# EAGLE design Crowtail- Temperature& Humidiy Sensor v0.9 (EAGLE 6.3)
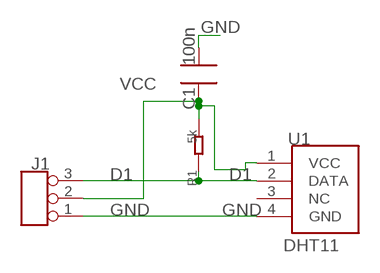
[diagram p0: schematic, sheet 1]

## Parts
C1  100n  C0603  [0603]
J1  TINKER_3P_DIP  [3P_2.0_DIP]
R1  5k  R0603  [0603]
U1  DHT11  [DHT11]

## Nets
D1: J1.3 R1.1 U1.2(DATA)
GND: C1.2 J1.1 U1.4(GND)
VCC: C1.1 J1.2 R1.2 U1.1(VCC)
Unconnected: U1.3(NC)

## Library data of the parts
C1 = CPT_SMD:C0603; C0603: 100N
J1 = Connector:TINKER_3P_DIP
R1 = CPT_SMD:R0603
U1 = Sensors:DHT11

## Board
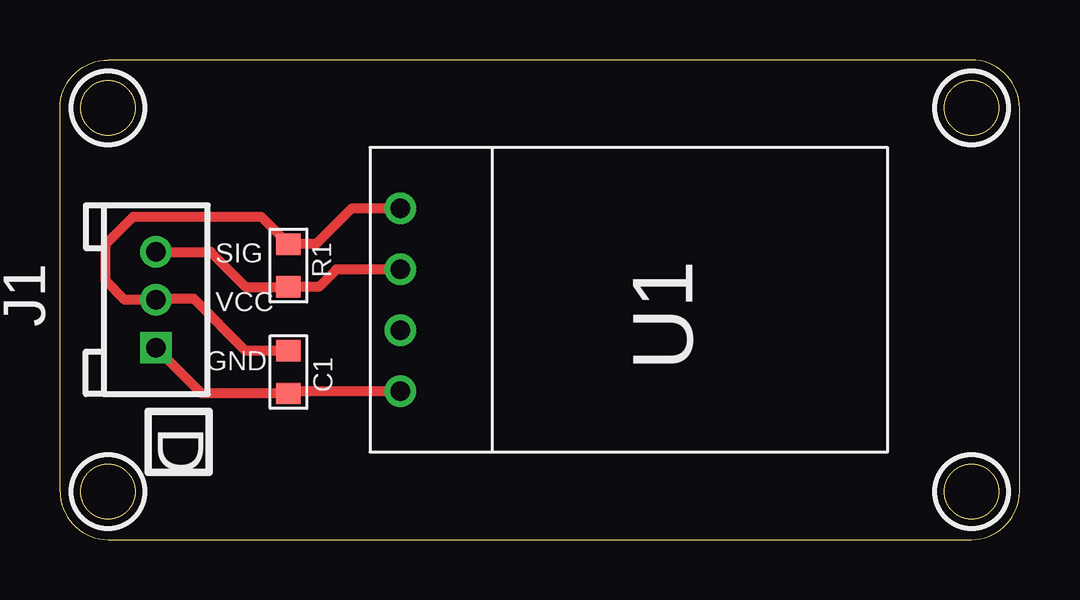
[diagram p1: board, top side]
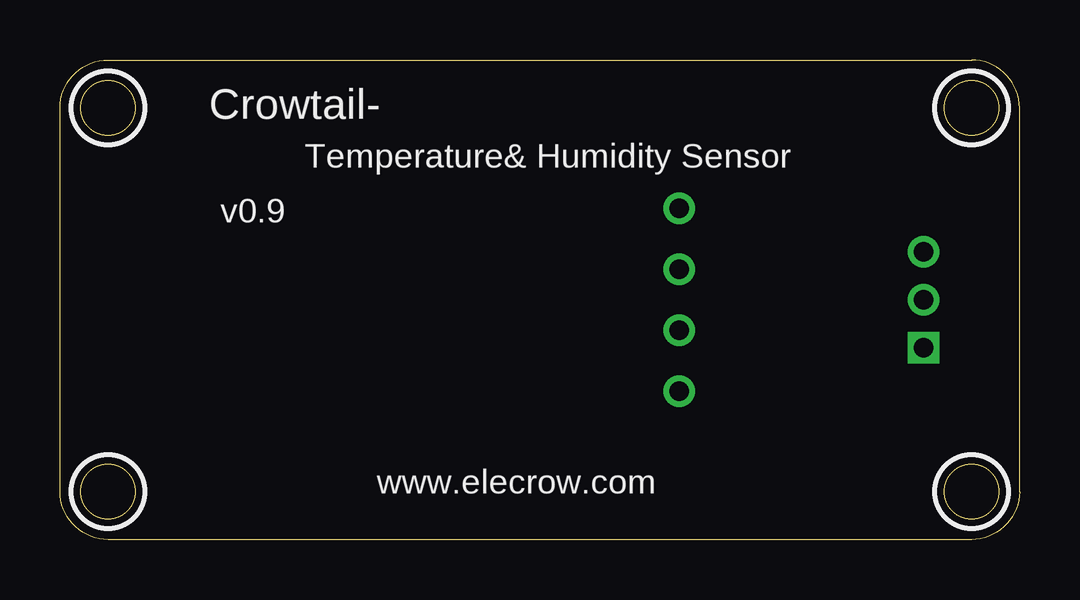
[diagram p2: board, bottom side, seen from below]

Size 40 x 20 mm. Coordinates in mm from the lower left corner, seen from the top.
Outline: 0,2 0,18 arc-90 2,20 38,20 arc-90 40,18 40,2 arc-90 38,0 2,0 arc-90 0,2
Outline: circle at 2,18 radius 1.14
Outline: circle at 2,2 radius 1.14
Outline: circle at 38,18 radius 1.14
Outline: circle at 38,2 radius 1.14
Copper layers (1*16): Top 0.035mm / dielectric 1.5mm / Bottom 0.035mm
Design rules "default": minimum track width 10mil, minimum drill 24mil, track to track 8mil, track to pad 8mil, pad to pad 8mil, via to via 8mil, smd to smd 8mil, copper to edge 40mil, drill to drill 8mil, minimum pad ring 10mil, minimum via ring 8mil, stop-mask expansion 4mil, vias tented up to drill 0mil, thermal gap 10mil
tRestrict: area 0.5,16.5 to 3.5,19.5; area 0.5,0.5 to 3.5,3.5; area 36.5,16.5 to 39.5,19.5; area 36.5,0.5 to 39.5,3.5
bRestrict: area 0.5,16.5 to 3.5,19.5; area 0.5,0.5 to 3.5,3.5; area 36.5,16.5 to 39.5,19.5; area 36.5,0.5 to 39.5,3.5

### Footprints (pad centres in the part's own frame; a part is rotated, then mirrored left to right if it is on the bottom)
0603 = smd 0.889 x 1.016: 1 -0.889,0; 2 0.889,0
3P_2.0_DIP = drill 0.8 pad 1.27 square: 1 -2,0 | drill 0.8 pad 1.27: 2 0,0; 3 2,0
DHT11 = drill 0.8: 1 -3.81,-3.81; 2 -1.27,-3.81; 3 1.27,-3.81; 4 3.81,-3.81

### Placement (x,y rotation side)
C1  9.53,6.99 270 top
J1  4,10 90 top
R1  9.53,11.43 90 top
U1  18,10 270 top

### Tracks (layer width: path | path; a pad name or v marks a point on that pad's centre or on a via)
D1
  Top 0.406: J1.3 6.29,12 7.75,10.54 R1.1 10.79,10.54 11.52,11.27 U1.2
GND
  Top 0.406: J1.1 5.9,6.1 C1.2 9.62,6.19 U1.4
VCC
  Top 0.406: U1.1 12.16,13.81 10.67,12.32 R1.2 8.38,13.46 3.05,13.46 1.91,12.32 1.91,10.79 2.7,10 J1.2 4.03,10.03 5.59,10.03 7.75,7.87 C1.1

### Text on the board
tPlace: SIG | VCC | GND | D
bPlace: Crowtail- | Temperature& Humidity Sensor | v0.9 | www.elecrow.com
